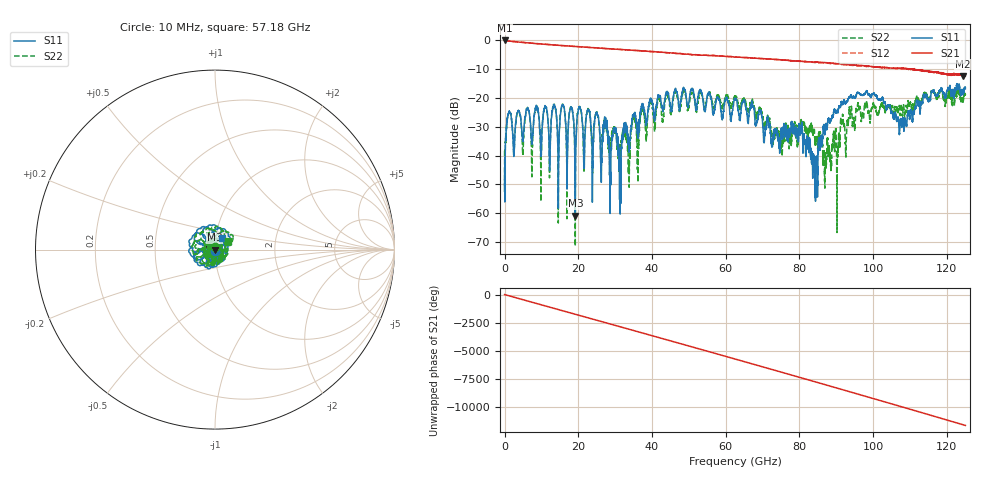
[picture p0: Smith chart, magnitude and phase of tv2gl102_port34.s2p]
!Keysight Technologies,N5247B,MY58422656,A.13.80.08
!Posted to IEEE NEA 05/29  by John Calvin
!Date: Thursday, July 29, 2021 13:51:29
!Correction: S11(Full 2 Port(1,2))
!S21(Full 2 Port(1,2))
!S12(Full 2 Port(1,2))
!S22(Full 2 Port(1,2))
!S2P File: Measurements: S11, S21, S12, S22:
# Hz S  dB  R 50
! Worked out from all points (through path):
!   12500 points, 10 MHz to 125 GHz, reference 50 ohm
!   highest |S21| = -0.03 dB at 50 MHz (marker M1); lowest = -12.4 dB at 124.3 GHz (marker M2)
!   lowest |S11| = -60.8 dB at 19.19 GHz (marker M3), VSWR 1.00, Z = 50 - j0.0862 ohm
!   |S11| at or under -10 dB: start of sweep to end of sweep
!   |S22| runs from -71.4 to -16.7 dB; largest |S21 - S12| = 0.071
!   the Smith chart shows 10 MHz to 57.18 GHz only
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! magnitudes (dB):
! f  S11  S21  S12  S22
! 10 MHz  -44.4  0.0  -0.1  -38.3
! 50 MHz  -48.4  0.0  -0.1  -49.0
! 1.27 GHz  -24.5  -0.3  -0.3  -24.7
! 7.42 GHz  -35.9  -1.0  -1.0  -46.7
! 8.68 GHz  -23.1  -1.1  -1.1  -22.9
! 9.86 GHz  -39.8  -1.2  -1.2  -55.9
! 13.43 GHz  -22.6  -1.6  -1.6  -22.3
! 14.6 GHz  -51.9  -1.7  -1.7  -47.7
! 15.8 GHz  -22.4  -1.8  -1.8  -22.3
! 19.19 GHz  -60.8  -2.1  -2.1  -54.0
! 20.85 GHz  -24.9  -2.3  -2.3  -25.4
! 29.92 GHz  -31.5  -3.0  -3.0  -31.9
! 31.16 GHz  -43.5  -3.1  -3.1  -36.5
! 41.68 GHz  -19.2  -4.1  -4.1  -20.4
! 62.51 GHz  -20.5  -5.8  -5.8  -18.9
! 74.94 GHz  -32.2  -6.7  -6.7  -36.8
! 83.34 GHz  -39.9  -7.5  -7.6  -29.9
! 86.84 GHz  -31.7  -7.7  -7.9  -47.6
! 93.7 GHz  -19.6  -8.5  -8.6  -26.1
! 104.2 GHz  -22.6  -9.5  -9.6  -22.7
! 124.3 GHz  -17.9  -12.4  -11.9  -20.2
! 125 GHz  -16.7  -12.3  -12.3  -18.6
